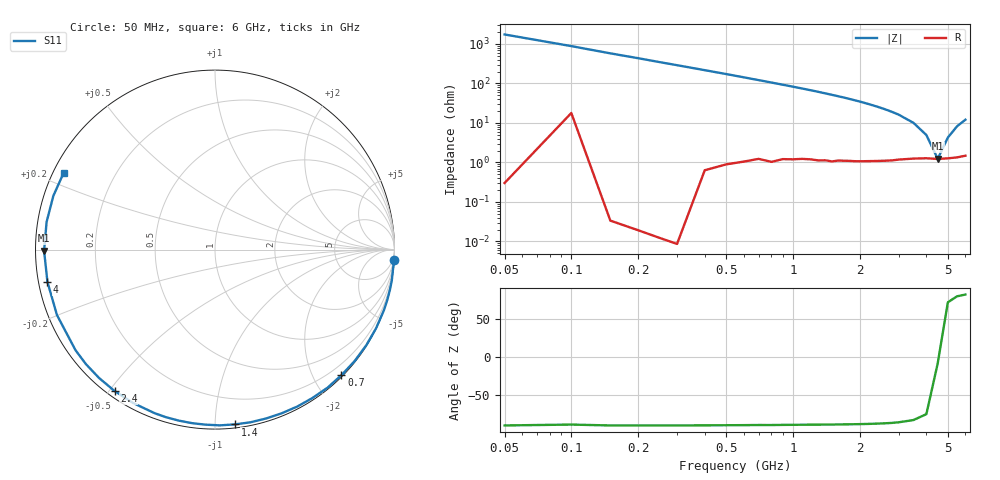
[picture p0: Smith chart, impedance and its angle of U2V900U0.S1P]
! SIEMENS Discrete & RF Semiconductors
! BBY52-02W
! Si Tuning Diode in SCD-80
! VR = 0.9 V
! S-Parameters:  September  1997
# GHz  S  MA  R  50
!  f  S11
! GHz  MAG  ANG
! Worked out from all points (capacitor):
!   34 points, 50 MHz to 6 GHz, reference 50 ohm
!   read as one part to ground: C = 1.83 pF near 50 MHz
!   lowest |Z| = 1.24 ohm at 4.5 GHz (marker M1)
!   series resonance near 4.521 GHz, so ESL is about 680 pH
!   S11 on the Smith chart (normalised r, x): 50 MHz: 0, -35; 700 MHz: 0.02, -2.43; 1.4 GHz: 0.02, -1.12; 2.4 GHz: 0.02, -0.52; 4 GHz: 0.03, -0.10; 6 GHz: 0.03, +0.24
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0.05  1 -3.3
0.2  1 -13.1
0.3  1 -19.6
0.4  0.9987 -26.0
0.5  0.9972 -32.3
0.6  0.9954 -38.6
0.7  0.9929 -44.8
0.8  0.9924 -50.8
0.9  0.9891 -56.7
1  0.9873 -62.3
1.1  0.9848 -67.8
1.3  0.9822 -78.4
1.4  0.9801 -83.5
1.5  0.9796 -88.4
1.6  0.9768 -93.1
1.8  0.9739 -102.0
2  0.9716 -110.3
2.2  0.9687 -118.2
2.4  0.9663 -125.4
2.6  0.9638 -132.1
2.8  0.9614 -138.4
3  0.9582 -144.2
3.5  0.953 -157.5
4  0.9507 -169.1
4.5  0.9523 -179.6
5  0.9508 170.7
5.5  0.9492 161.6
6  0.9456 153.1
